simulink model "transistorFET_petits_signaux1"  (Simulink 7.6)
settings: Solver=ode15s  StartTime=0.0  StopTime=0.06  RelTol=1e-3
InitFcn:
  | clc
  | rho=1e6;
  | RD=1000;
  | RG1=47e3;
  | RG2=47e3;
  | RG=RG1*RG2/(RG1+RG2);
  | g=3000e-6;
StopFcn:
  | close all
  | load es.mat
  | plot(x(1,:),x(2,:),x(1,:),x(3,:))
  | title('Signaux d''E/S - Schéma équivalent du transistor FET')
  | xlabel('temps')
  | grid
libraries: fl_lib x11, nesl_utility x3

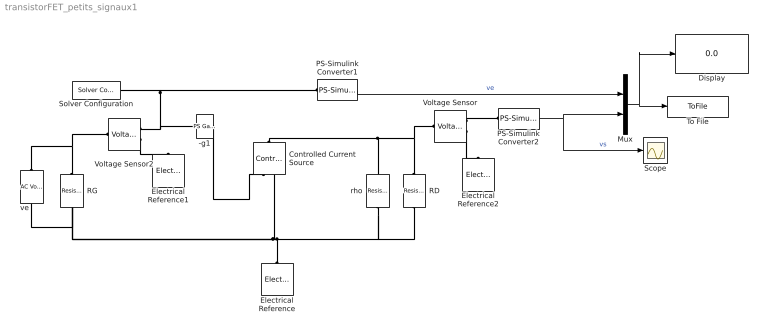
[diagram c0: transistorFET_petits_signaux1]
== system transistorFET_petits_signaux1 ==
  -g1 : fl_lib/Physical Signals/Functions/PS Gain  DialogController=NetworkEngine.DynNeDlgSource  SystemSampleTime=-1  gain=-g  LocalVarLogging=[]
  Controlled Current Source : fl_lib/Electrical/Electrical Sources/Controlled Current Source  DialogController=NetworkEngine.DynNeDlgSource  SystemSampleTime=-1  i_Log=off  v_Log=off  LocalVarNames=|i|v  LocalVarDescs=|i|v  LocalVarLogging=[0 0]
  Display : Display
  Electrical Reference : fl_lib/Electrical/Electrical Elements/Electrical Reference  DialogController=NetworkEngine.DynNeDlgSource  SystemSampleTime=-1  i_Log=off  LocalVarNames=|i  LocalVarDescs=|i  LocalVarLogging=0
  Electrical Reference1 : fl_lib/Electrical/Electrical Elements/Electrical Reference  DialogController=NetworkEngine.DynNeDlgSource  SystemSampleTime=-1  i_Log=off  LocalVarNames=|i  LocalVarDescs=|i  LocalVarLogging=0
  Electrical Reference2 : fl_lib/Electrical/Electrical Elements/Electrical Reference  DialogController=NetworkEngine.DynNeDlgSource  SystemSampleTime=-1  i_Log=off  LocalVarNames=|i  LocalVarDescs=|i  LocalVarLogging=0
  Mux : Mux  Inputs=2
  PS-Simulink Converter1 : nesl_utility/PS-Simulink Converter  DialogController=NetworkEngine.DynNeUtilDlgSource  SystemSampleTime=-1  PhysicalDomain=network_engine_domain  LeftPortType=input  RightPortType=output  SubClassName=ps_output  Unit=1  AffineConversion=off
  PS-Simulink Converter2 : nesl_utility/PS-Simulink Converter  DialogController=NetworkEngine.DynNeUtilDlgSource  SystemSampleTime=-1  PhysicalDomain=network_engine_domain  LeftPortType=input  RightPortType=output  SubClassName=ps_output  Unit=1  AffineConversion=off
  RD : fl_lib/Electrical/Electrical Elements/Resistor  DialogController=NetworkEngine.DynNeDlgSource  SystemSampleTime=-1  R=RD Ohm  i_Log=off  v_Log=off  LocalVarNames=|i|v  LocalVarDescs=|i|v  LocalVarLogging=[0 0]
  RG : fl_lib/Electrical/Electrical Elements/Resistor  DialogController=NetworkEngine.DynNeDlgSource  SystemSampleTime=-1  R=RG Ohm  i_Log=off  v_Log=off  LocalVarNames=|i|v  LocalVarDescs=|i|v  LocalVarLogging=[0 0]
  Scope : Scope
  Solver Configuration : nesl_utility/Solver Configuration  DialogController=NetworkEngine.DynNeUtilDlgSource  SystemSampleTime=-1  PhysicalDomain=network_engine_domain  LeftPortType=input  RightPortType=generic  SubClassName=solver  Accelerate=off  Profile=off  ResidualTolerance=1e-9  MaxNonlinIter=3  MaxModeIter=2  DoFixedCost=off  UseLocalSampling=off  DoDC=off  LinearAlgebra=Sparse  LocalSolverSampleTime=.001  LocalSolverChoice=NE_BACKWARD_EULER_ADVANCER  UseLocalSolver=off
  To File : ToFile  Filename=es.mat  MatrixName=x
  Voltage Sensor : fl_lib/Electrical/Electrical Sensors/Voltage Sensor  DialogController=NetworkEngine.DynNeDlgSource  SystemSampleTime=-1  i1_Log=off  v1_Log=off  LocalVarNames=|i1|v1  LocalVarDescs=|i1|v1  LocalVarLogging=[0 0]
  Voltage Sensor2 : fl_lib/Electrical/Electrical Sensors/Voltage Sensor  DialogController=NetworkEngine.DynNeDlgSource  SystemSampleTime=-1  i1_Log=off  v1_Log=off  LocalVarNames=|i1|v1  LocalVarDescs=|i1|v1  LocalVarLogging=[0 0]
  rho : fl_lib/Electrical/Electrical Elements/Resistor  DialogController=NetworkEngine.DynNeDlgSource  SystemSampleTime=-1  R=rho Ohm  i_Log=off  v_Log=off  LocalVarNames=|i|v  LocalVarDescs=|i|v  LocalVarLogging=[0 0]
  ve : fl_lib/Electrical/Electrical Sources/AC Voltage Source  DialogController=NetworkEngine.DynNeDlgSource  SystemSampleTime=-1  amp=10 mV  shift=0 rad  omega=60 Hz  i_Log=off  v_Log=off  LocalVarNames=|i|v  LocalVarDescs=|i|v  LocalVarLogging=[0 0]
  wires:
  PS-Simulink Converter2/1 -> Mux/2, Scope/1  "vs"
  PS-Simulink Converter1/1 -> Mux/1  "ve"
  Mux/1 -> To File/1, Display/1
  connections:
  RG/RConn1 -- Voltage Sensor2/LConn1 -- ve/LConn1
  Voltage Sensor2/RConn2 -- Electrical Reference1/LConn1
  Voltage Sensor2/RConn1 -- PS-Simulink Converter1/LConn1 -- Solver Configuration/RConn1 -- -g1/LConn1
  RD/RConn1 -- rho/RConn1 -- Controlled Current Source/LConn1 -- Voltage Sensor/LConn1
  Voltage Sensor/RConn2 -- Electrical Reference2/LConn1
  Voltage Sensor/RConn1 -- PS-Simulink Converter2/LConn1
  RG/LConn1 -- ve/RConn1 -- rho/LConn1 -- RD/LConn1 -- Controlled Current Source/RConn2 -- Electrical Reference/LConn1
  -g1/RConn1 -- Controlled Current Source/RConn1
